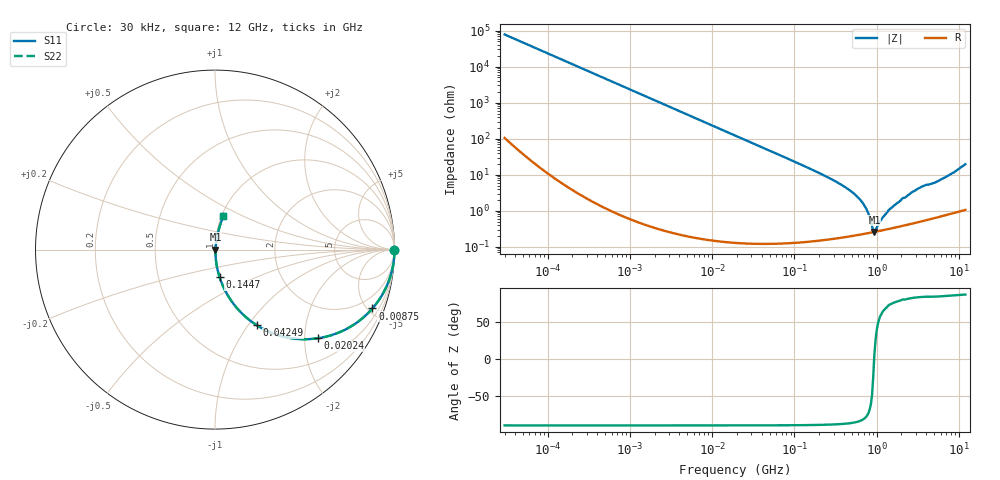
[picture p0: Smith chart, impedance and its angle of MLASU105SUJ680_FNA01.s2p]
! MLASU105SUJ680_FNA01  S-PARAMETER MODEL  ( General Type )
! Model Generated by TAIYO YUDEN Corporation (http://www.ty-top.com)
! Version 4.0
! TAIYO YUDEN Control No. 120810
! Copyright(c) 2003 TAIYO YUDEN CO.,LTD. All Rights Reserved.
! Product Description (link to TY-COMPAS)
! https://ds.yuden.co.jp/TYCOMPAS/or/detail?pn=MLASU105SUJ680JFNA01&u=M
! Products Name : Multilayer Ceramic Capacitors
! Characteristics :
!  Capacitance : 68 pF , Rated Voltage : 50V , TCC : UJ / U2J
!  Case Size : 1.0 x 0.5 / 0.039 x 0.02 [mm/inch] , Thickness : 0.5 / 0.02 [mm/inch]
!  (Conditions: Temperature = 25 degC , DC Bias Current/Voltage = 0A / 0V)
! External Node Assignments :
!  1  o---| |---o  2
! GND o---------o GND
! Frequency Range : 0.03MHz  -  12000MHz  [ 401 STEP ]
# MHz S RI R 50
! Freq[MHz].  S11 Real  S11 Imag  S21 Real  S21 Imag  S12 Real  S12 Imag  S22 Real  S22 Imag
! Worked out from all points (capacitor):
!   401 points, 30 kHz to 12 GHz, reference 50 ohm
!   read as one part in series: C = 67.9 pF near 32 kHz
!   lowest |Z| = 260 mohm at 939.2 MHz (marker M1)
!   series resonance near 933.4 MHz, so ESL is about 430 pH
!   S11 on the Smith chart (normalised r, x): 30 kHz: open; 8.75 MHz: 1.00, -5.35; 20.24 MHz: 1.00, -2.31; 42.49 MHz: 1.00, -1.10; 144.7 MHz: 1.00, -0.32; 12 GHz: 1.02, +0.39
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0.03  1 -0.00128  3.36e-06 0.00128  3.36e-06 0.00128  1 -0.00128
0.260295  0.9999 -0.0111  0.000127 0.0111  0.000127 0.0111  0.9999 -0.0111
2.258455  0.9908 -0.0955  0.00924 0.0955  0.00924 0.0955  0.9908 -0.0955
8.750395  0.8774 -0.3277  0.1226 0.3277  0.1226 0.3277  0.8774 -0.3277
18.97367  0.6035 -0.4886  0.3965 0.4886  0.3965 0.4886  0.6035 -0.4886
20.23772  0.5723 -0.4942  0.4277 0.4942  0.4277 0.4942  0.5723 -0.4942
42.48934  0.2329 -0.4216  0.7671 0.4216  0.7671 0.4216  0.2329 -0.4216
73.51358  0.0921 -0.2872  0.9079 0.2872  0.9079 0.2872  0.0921 -0.2872
144.7024  0.0256 -0.1537  0.9744 0.1537  0.9744 0.1537  0.0256 -0.1537
164.6252  0.02 -0.1349  0.98 0.1349  0.98 0.1349  0.02 -0.1349
356.9603  0.00486 -0.0556  0.9951 0.0556  0.9951 0.0556  0.00486 -0.0556
560.6502  0.00278 -0.0265  0.9972 0.0265  0.9972 0.0265  0.00278 -0.0265
725.66  0.00246 -0.0126  0.9975 0.0126  0.9975 0.0126  0.00246 -0.0126
799.3715  0.00246 -0.00766  0.9975 0.00766  0.9975 0.00766  0.00246 -0.00766
880.5704  0.00251 -0.00279  0.9975 0.00279  0.9975 0.00279  0.00251 -0.00279
939.2353  0.00258 0.000271  0.9974 -0.000271  0.9974 -0.000271  0.00258 0.000271
970.0175  0.00262 0.00122  0.9974 -0.00122  0.9974 -0.00122  0.00262 0.00122
1139.739  0.00284 0.00489  0.9972 -0.00489  0.9972 -0.00489  0.00284 0.00489
1428.372  0.00325 0.0103  0.9968 -0.0103  0.9968 -0.0103  0.00325 0.0103
2903.719  0.00579 0.0352  0.9942 -0.0352  0.9942 -0.0352  0.00579 0.0352
5534.236  0.0107 0.0644  0.9893 -0.0644  0.9893 -0.0644  0.0107 0.0644
12000  0.0464 0.1851  0.9536 -0.1851  0.9536 -0.1851  0.0464 0.1851
